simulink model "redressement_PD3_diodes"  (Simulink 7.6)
settings: Solver=ode23tb  StartTime=0.0  StopTime=0.05  RelTol=1e-3
InitFcn:
  | clc
StopFcn:
  | close all, clc, clear all
  | load signaux_phases.mat
  | plot(x(1,:),x(2,:),x(1,:),x(3,:),x(1,:),x(4,:))
  | 
  | grid
  | title('Tensions aux anodes vA, cathodes vK et de sortie vK-vA')
  | xlabel('temps')
libraries: powerlib x18, powerlib_extras x2

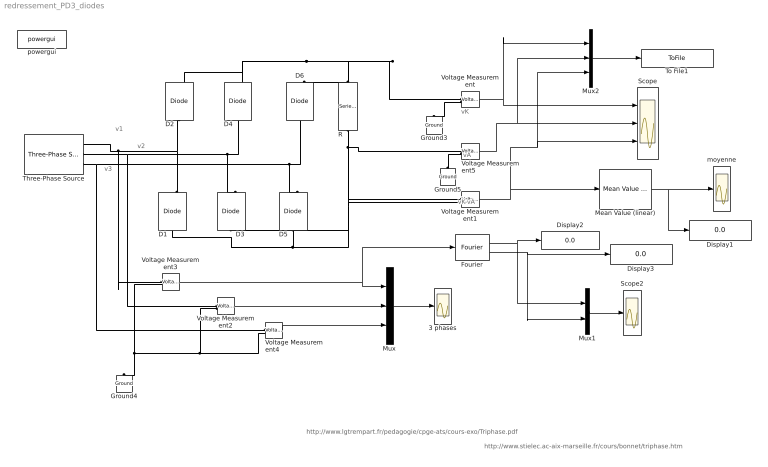
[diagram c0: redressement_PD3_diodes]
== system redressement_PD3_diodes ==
  note: http://www.lgtrempart.fr/pedagogie/cpge-ats/cours-exo/Triphase.pdf
  note: http://www.stielec.ac-aix-marseille.fr/cours/bonnet/triphase.htm
  note: vK
  note: vA
  note: vK-vA
  note: v1
  note: v2
  note: v3
  3 phases : Scope
  D{1..6} (6 alike) : powerlib/Power Electronics/Diode  DialogController=POWERSYS.PowerSysDialog  SystemSampleTime=-1  Ron=0.001  Lon=0  Vf=0.8  IC=0  UseSnubber=off  Rs=500  Cs=250e-9  Measurements=on
  Display1 : Display
  Display2 : Display
  Display3 : Display
  Fourier : powerlib_extras/Measurements/Fourier  DialogController=POWERSYS.PowerSysDialog  SystemSampleTime=-1  f1=60  n=1
  Ground3 : powerlib/Elements/Ground  DialogController=POWERSYS.PowerSysDialog  PhysicalDomain=powersysdomain  SubClassName=unknown  LeftPortType=p1  RightPortType=p1  LConnTagsString=a
  Ground4 : powerlib/Elements/Ground  DialogController=POWERSYS.PowerSysDialog  PhysicalDomain=powersysdomain  SubClassName=unknown  LeftPortType=p1  RightPortType=p1  LConnTagsString=a
  Ground5 : powerlib/Elements/Ground  DialogController=POWERSYS.PowerSysDialog  PhysicalDomain=powersysdomain  SubClassName=unknown  LeftPortType=p1  RightPortType=p1  LConnTagsString=a
  Mean Value (linear) : powerlib_extras/Measurements/Mean Value (linear)  DialogController=POWERSYS.PowerSysDialog  SystemSampleTime=-1  Freq=60  n=3  Vinit=0
  Mux : Mux  Inputs=3
  Mux1 : Mux  Inputs=2
  Mux2 : Mux  Inputs=3
  R : powerlib/Elements/Series RLC Branch  DialogController=POWERSYS.PowerSysDialog  PhysicalDomain=powersysdomain  SubClassName=unknown  LeftPortType=p1  RightPortType=p1  LConnTagsString=__new0  RConnTagsString=__new0  BranchType=R  Resistance=2  Inductance=1e-3  SetiL0=off  InitialCurrent=0  Capacitance=1e-6  Setx0=off  InitialVoltage=0  Measurements=None
  Scope : Scope  NumInputPorts=3
  Scope2 : Scope
  Three-Phase Source : powerlib/Electrical Sources/Three-Phase Source  DialogController=POWERSYS.PowerSysDialog  SystemSampleTime=-1  Voltage=380  PhaseAngle=0  Frequency=60  InternalConnection=Yg  SpecifyImpedance=on  Resistance=0.8929  Inductance=16.58e-3  ShortCircuitLevel=100e6  BaseVoltage=25e3  XRratio=7
  To File1 : ToFile  Filename=signaux_phases  MatrixName=x
  Voltage Measurement{,1..5} (6 alike) : powerlib/Measurements/Voltage Measurement  DialogController=POWERSYS.PowerSysDialog  SystemSampleTime=-1  PhasorSimulation=off  OutputType=Complex  PSBequivalent=0
  moyenne : Scope
  powergui : powerlib/powergui  SystemSampleTime=-1  SimulationMode=Continuous  SampleTime=0  frequency=60  SPID=off  DisableSnubberDevices=off  DisableRonSwitches=off  DisableVfSwitches=off  SwTol=0  Interpol=off  frequencyindice=0  echomessages=off  HookPort=off  DisplayEquations=off  FunctionMessages=off  EnableUseOfTLC=off  x0status=blocks  RestoreLinks=warning  ResistiveCurrentMeasurement=off  Frange=[0:2:500]  Ylog=off  Xlog=on  ShowGrid=off  save=off  variable=ZData  ZoomFFT=on  StartTime=0.0  cycles=1  DisplayStyle=1  fundamental=60  FreqAxis=off  MaxFrequency=1000  frequencyindicesteady=60  RmsSteady=1  display=off  Ts=0  methode=off
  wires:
  Fourier/1 -> Display2/1, Mux1/1
  Voltage Measurement4/1 -> Mux/3
  Voltage Measurement2/1 -> Mux/2
  Voltage Measurement3/1 -> Fourier/1, Mux/1
  Fourier/2 -> Display3/1, Mux1/2
  Voltage Measurement/1 -> Scope/1, Mux2/1
  Voltage Measurement5/1 -> Scope/2, Mux2/2
  Voltage Measurement1/1 -> Scope/3, Mux2/3, Mean Value (linear)/1
  Mux/1 -> 3 phases/1
  Mux1/1 -> Scope2/1
  Mux2/1 -> To File1/1
  Mean Value (linear)/1 -> moyenne/1, Display1/1
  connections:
  Three-Phase Source/RConn3 -- D6/LConn1 -- D5/RConn1 -- Voltage Measurement4/LConn1
  D1/LConn1 -- D3/LConn1 -- D5/LConn1 -- Voltage Measurement5/LConn1 -- R/LConn1 -- Voltage Measurement1/LConn2
  Voltage Measurement/LConn1 -- Voltage Measurement1/LConn1 -- D2/RConn1 -- D4/RConn1 -- D6/RConn1 -- R/RConn1
  Voltage Measurement2/LConn2 -- Voltage Measurement3/LConn2 -- Ground4/LConn1 -- Voltage Measurement4/LConn2
  Voltage Measurement/LConn2 -- Ground3/LConn1
  Ground5/LConn1 -- Voltage Measurement5/LConn2
  D1/RConn1 -- Three-Phase Source/RConn1 -- Voltage Measurement3/LConn1 -- D2/LConn1
  Three-Phase Source/RConn2 -- D4/LConn1 -- D3/RConn1 -- Voltage Measurement2/LConn1
